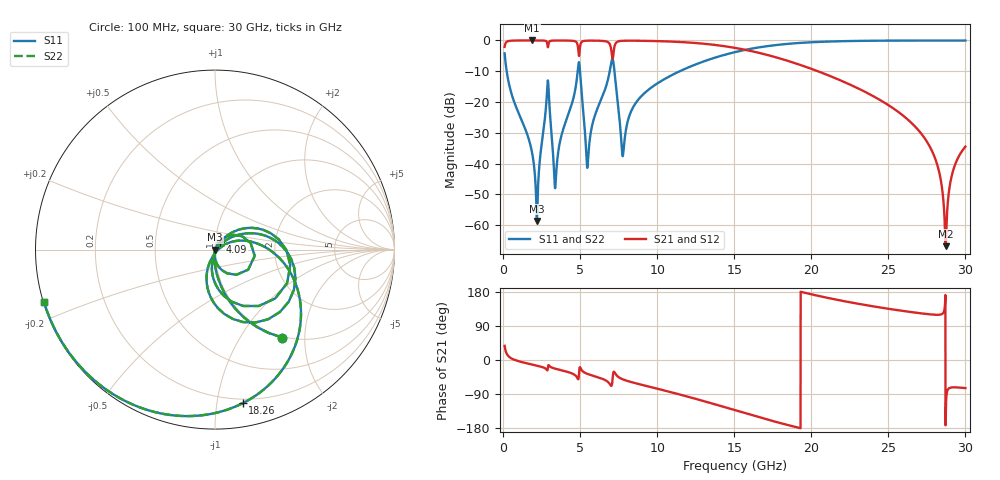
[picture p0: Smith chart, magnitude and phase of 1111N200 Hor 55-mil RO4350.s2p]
# GHz S MA R 50
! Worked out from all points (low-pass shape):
!   3201 points, 100 MHz to 30 GHz, reference 50 ohm
!   highest |S21| = -0.01 dB at 1.885 GHz (marker M1); lowest = -66.9 dB at 28.72 GHz (marker M2)
!   |S21| within 3 dB of the highest: start of sweep to 4.882 GHz; 7.193 GHz to 15.68 GHz (8.484 GHz wide, 74.2 % of centre)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
!   lowest |S11| = -58.7 dB at 2.193 GHz (marker M3), VSWR 1.00, Z = 50.1 - j0.0431 ohm
!   |S11| at or under -10 dB: 233.6 MHz to 4.842 GHz (4.609 GHz wide, 182 % of centre); 4.991 GHz to 6.922 GHz (1.931 GHz wide, 32.4 % of centre); 7.227 GHz to 11.47 GHz (4.243 GHz wide, 45.4 % of centre)
!   |S22| runs from -58.7 to 0.0 dB; largest |S21 - S12| = 0
!   S11 on the Smith chart (normalised r, x): 100 MHz: 0.98, -1.55; 4.09 GHz: 1.05, +0.09; 18.26 GHz: 0.17, -1.18; 30 GHz: 0.00, -0.15
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0.1  0.6168 -52.6  0.7869 37.4  0.7869 37.4  0.6168 -52.6
1.884656  0.01488 -98.7  0.9988 -12.0  0.9988 -12.0  0.01488 -98.7
2.193  0.001165 -21.7  0.9986 -14.9  0.9986 -14.9  0.001165 -21.7
2.86575  0.1688 25.9  0.8892 -27.2  0.8892 -27.2  0.1688 25.9
3.389  0.004096 -2.4  0.9958 -23.0  0.9958 -23.0  0.004096 -2.4
4.089781  0.04966 56.0  0.9951 -30.4  0.9951 -30.4  0.04966 56.0
4.865312  0.36 9.0  0.7684 -50.7  0.7684 -50.7  0.36 9.0
5.089563  0.1477 -94.9  0.9366 -26.1  0.9366 -26.1  0.1477 -94.9
5.491344  0.009561 -3.1  0.9914 -36.9  0.9914 -36.9  0.009561 -3.1
7.05175  0.4756 -19.5  0.6142 -66.9  0.6142 -66.9  0.4756 -19.5
7.780563  0.01353 -28.5  0.9866 -51.2  0.9866 -51.2  0.01353 -28.5
8.462656  0.08411 26.3  0.9899 -59.9  0.9899 -59.9  0.08411 26.3
10.06978  0.2047 12.5  0.9738 -76.4  0.9738 -76.4  0.2047 12.5
15.05  0.6454 -43.0  0.7566 -132.5  0.7566 -132.5  0.6454 -43.0
18.26425  0.8696 -79.8  0.4837 -169.4  0.4837 -169.4  0.8696 -79.8
20.03956  0.9347 -97.4  0.343 173.0  0.343 173.0  0.9347 -97.4
25.01978  0.9926 -135.6  0.08833 135.1  0.08833 135.1  0.9926 -135.6
27.76684  0.9965 -151.6  0.0173 120.2  0.0173 120.2  0.9965 -151.6
28.32747  0.9966 -154.6  0.006745 119.6  0.006745 119.6  0.9966 -154.6
28.71991  0.9967 -156.7  0.000454 -153.2  0.000454 -153.2  0.9967 -156.7
29.18709  0.9966 -159.1  0.007445 -72.2  0.007445 -72.2  0.9966 -159.1
30  0.9965 -163.1  0.01882 -74.1  0.01882 -74.1  0.9965 -163.1
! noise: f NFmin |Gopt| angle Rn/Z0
0.1  0.0007001  0.7487  2.603  0.0005607
3.417  0.01516  0.6302  23.06  0.007404
6.743  0.05537  0.787  44.15  0.04605
10.06  0.02756  0.4875  61.26  0.007103
13.39  0.03658  0.5096  75.29  0.00864
16.7  0.05496  0.6075  90.52  0.01362
20.03  0.09371  0.7398  108.3  0.0258
23.35  0.1961  0.8661  127.4  0.063
26.67  0.6942  0.96  146  0.3372
30  1.526  0.9811  163  0.4123
